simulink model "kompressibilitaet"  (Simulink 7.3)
settings: Solver=ode23tb  StartTime=0.0  StopTime=1000  MaxStep=0.5  RelTol=1e-3
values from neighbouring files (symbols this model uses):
  c_d = 0.9658    [dynamic_main.m]    (also in Parameter.m = 1; Parameter_sim.m; static_main.m = inv(H3'*H3)*H3'*y3)
  d_F = 2    [dynamic_main.m]    (also in Parameter.m; Parameter_sim.m; static_main.m)
  g = 9.81    [dynamic_main.m]    (also in Parameter.m; Parameter_sim.m; static_main.m)
  h_W0 = 390    [dynamic_main.m]    (also in Parameter.m; Parameter_sim.m; static_main.m)
  l_F = 741    [dynamic_main.m]    (also in Parameter.m; Parameter_sim.m; static_main.m)
  p_0 = 0    [dynamic_main.m]    (also in Parameter.m; Parameter_sim.m; static_main.m)
  rho = 1000    [dynamic_main.m]    (also in Parameter.m; Parameter_sim.m; static_main.m)
  sigma_0 = fminsearch(@(sigma_0)err_kompressibilitaet(sigma_0,time_bb,V_flw_F_bb,p_F_bb,x_bb),sigma_0_0)    [dynamic_main.m]    (also in Parameter.m = 1e-15; Parameter_sim.m = 6.279e-10)
  V_F_IC = l_F*pi*d_F^2/4    (= 2327.92015631)    [dynamic_main.m]    (also in Parameter.m; Parameter_sim.m; static_main.m)

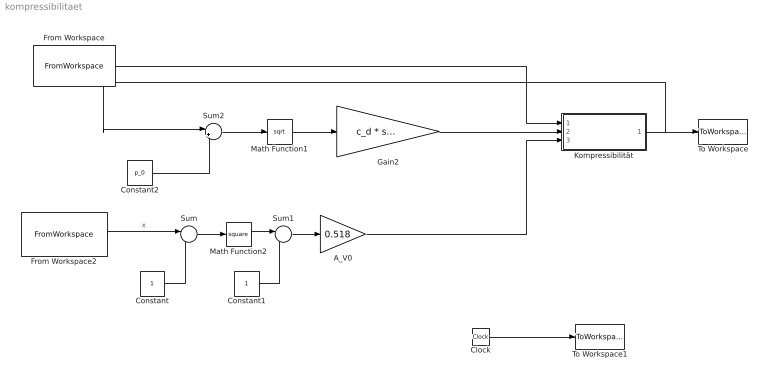
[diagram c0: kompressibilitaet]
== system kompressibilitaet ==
  A_V0 : Gain  Gain=0.518  ParameterDataType=sfix(16)  ParameterScaling=2^0  OutDataType=sfix(16)  OutScaling=2^0
  Clock : Clock
  Constant : Constant  OutDataType=sfix(16)  OutScaling=2^0
  Constant1 : Constant  OutDataType=sfix(16)  OutScaling=2^0
  Constant2 : Constant  Value=p_0  OutDataType=sfix(16)  OutScaling=2^0
  From Workspace : FromWorkspace  VariableName=[time_bb V_flw_F_bb]  SampleTime=0
  From Workspace2 : FromWorkspace  VariableName=[time_bb x_bb]  SampleTime=0
  Gain2 : Gain  Gain=c_d * sqrt(2/rho)  ParameterDataType=sfix(16)  ParameterScaling=2^0  OutDataType=sfix(16)  OutScaling=2^0
  Kompressibilität : Subsystem
  Math Function1 : Math  Operator=sqrt  OutDataType=sfix(16)  OutScaling=2^0
  Math Function2 : Math  Operator=square  OutDataType=sfix(16)  OutScaling=2^0
  Sum : Sum  Inputs=|-+  OutDataType=sfix(16)  OutScaling=2^0
  Sum1 : Sum  Inputs=|-+  OutDataType=sfix(16)  OutScaling=2^0
  Sum2 : Sum  Inputs=|+-  OutDataType=sfix(16)  OutScaling=2^0
  To Workspace : ToWorkspace  VariableName=p_F  SampleTime=-1  SaveFormat=Array
  To Workspace1 : ToWorkspace  VariableName=time_sim  SampleTime=-1  SaveFormat=Array
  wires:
  From Workspace/1 -> Kompressibilität/1(V_flw_F)
  Clock/1 -> To Workspace1/1
  Kompressibilität/1(p_F) -> To Workspace/1, Sum2/1
  From Workspace2/1 -> Sum/1  "x"
  Constant/1 -> Sum/2
  Sum/1 -> Math Function2/1
  Constant1/1 -> Sum1/2
  Sum1/1 -> A_V0/1
  Math Function2/1 -> Sum1/1
  A_V0/1 -> Kompressibilität/3(A_V)
  Constant2/1 -> Sum2/2
  Sum2/1 -> Math Function1/1
  Math Function1/1 -> Gain2/1
  Gain2/1 -> Kompressibilität/2(v_V)

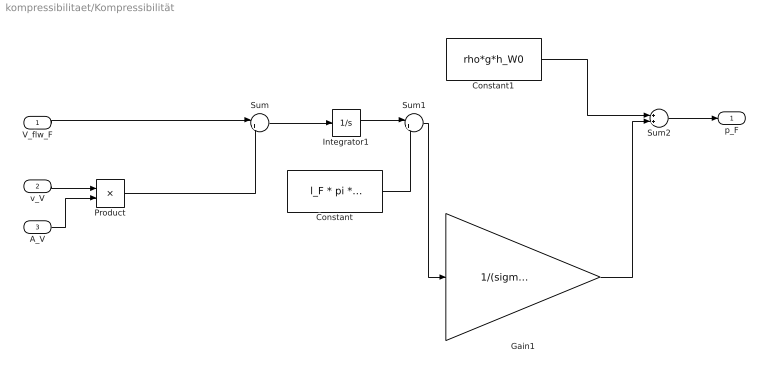
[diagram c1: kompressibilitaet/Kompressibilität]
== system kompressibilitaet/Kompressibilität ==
  V_flw_F : Inport  OutDataType=sfix(16)  OutScaling=2^0
  v_V : Inport  Port=2  OutDataType=sfix(16)  OutScaling=2^0
  A_V : Inport  Port=3  OutDataType=sfix(16)  OutScaling=2^0
  Constant : Constant  Value=l_F * pi * d_F^2 / 4  OutDataType=sfix(16)  OutScaling=2^0
  Constant1 : Constant  Value=rho*g*h_W0  OutDataType=sfix(16)  OutScaling=2^0
  Gain1 : Gain  Gain=1/(sigma_0*l_F*pi*d_F^2/4)  ParameterDataType=sfix(16)  ParameterScaling=2^0  OutDataType=sfix(16)  OutScaling=2^0
  Integrator1 : Integrator  InitialCondition=V_F_IC
  Product : Product  OutDataType=sfix(16)  OutScaling=2^0
  Sum : Sum  Inputs=|+-  OutDataType=sfix(16)  OutScaling=2^0
  Sum1 : Sum  Inputs=|+-  OutDataType=sfix(16)  OutScaling=2^0
  Sum2 : Sum  OutDataType=sfix(16)  OutScaling=2^0
  p_F : Outport  OutDataType=sfix(16)  OutScaling=2^0
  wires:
  v_V/1 -> Product/1
  A_V/1 -> Product/2
  Product/1 -> Sum/2
  Sum/1 -> Integrator1/1
  Constant/1 -> Sum1/2
  Sum1/1 -> Gain1/1
  Integrator1/1 -> Sum1/1
  Gain1/1 -> Sum2/2
  Sum2/1 -> p_F/1
  Constant1/1 -> Sum2/1
  V_flw_F/1 -> Sum/1
